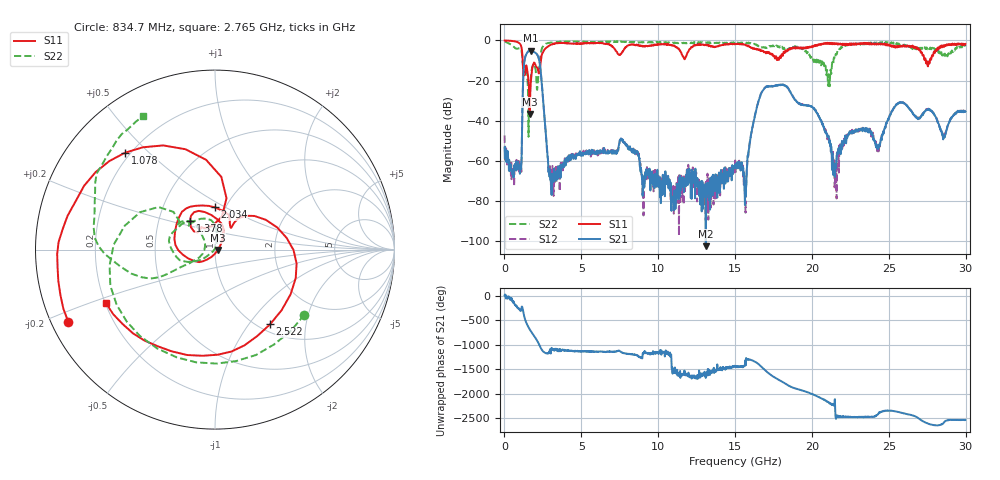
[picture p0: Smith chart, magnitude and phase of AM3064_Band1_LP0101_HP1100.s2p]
# Hz S DB R 50.0
!freq dBS11 angS11 dBS21 angS21 dBS12 angS12 dBS22 angS22
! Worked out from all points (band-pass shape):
!   1600 points, 10 MHz to 29.98 GHz, reference 50 ohm
!   highest |S21| = -5.04 dB at 1.697 GHz (marker M1); lowest = -102.5 dB at 13.09 GHz (marker M2)
!   |S21| within 3 dB of the highest: 1.361 GHz to 2.191 GHz (829.7 MHz wide, 46.7 % of centre)
!   lowest |S11| = -36.6 dB at 1.641 GHz (marker M3), VSWR 1.03, Z = 51.5 - j0.191 ohm
!   |S11| at or under -10 dB: 1.187 GHz to 2.366 GHz (1.18 GHz wide, 66.4 % of centre); 27.4 GHz to 27.68 GHz (281.5 MHz wide, 1.02 % of centre)
!   |S22| runs from -47.9 to -0.4 dB; largest |S21 - S12| = 0.0077
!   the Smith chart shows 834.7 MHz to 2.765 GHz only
!   S11 on the Smith chart (normalised r, x): 834.7 MHz: 0.05, -0.23; 1.078 GHz: 0.18, +0.42; 1.378 GHz: 0.72, +0.24; 2.034 GHz: 0.89, +0.44; 2.522 GHz: 1.12, -1.27; 2.765 GHz: 0.20, -0.22
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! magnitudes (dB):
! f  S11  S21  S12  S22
! 10 MHz  0.0  -53.5  -47.4  -0.4
! 834.7 MHz  -0.8  -64.3  -61.3  -4.2
! 1.078 GHz  -2.7  -64.1  -63.6  -4.5
! 1.378 GHz  -13.5  -7.6  -7.6  -14.0
! 1.641 GHz  -36.6  -5.1  -5.0  -24.3
! 1.697 GHz  -23.1  -5.0  -5.0  -19.6
! 2.034 GHz  -12.6  -6.3  -6.2  -15.0
! 2.522 GHz  -5.7  -30.1  -30.2  -2.9
! 2.765 GHz  -3.4  -53.0  -55.0  -1.5
! 3.121 GHz  -1.9  -66.3  -62.5  -1.0
! 5.015 GHz  -1.5  -56.6  -56.2  -0.7
! 7.657 GHz  -5.8  -50.0  -49.5  -0.7
! 10 GHz  -2.0  -72.9  -69.1  -0.9
! 13.09 GHz  -2.3  -102.5  -89.9  -1.0
! 15 GHz  -1.9  -61.6  -59.7  -1.5
! 15.68 GHz  -2.4  -72.2  -85.8  -1.3
! 16.99 GHz  -6.2  -23.3  -23.2  -3.5
! 19.99 GHz  -3.4  -33.1  -33.0  -9.3
! 21.45 GHz  -1.9  -61.5  -67.0  -8.5
! 25 GHz  -2.0  -39.1  -38.7  -1.2
! 28.58 GHz  -3.0  -48.2  -47.6  -7.4
! 29.98 GHz  -1.8  -35.5  -35.4  -2.9
